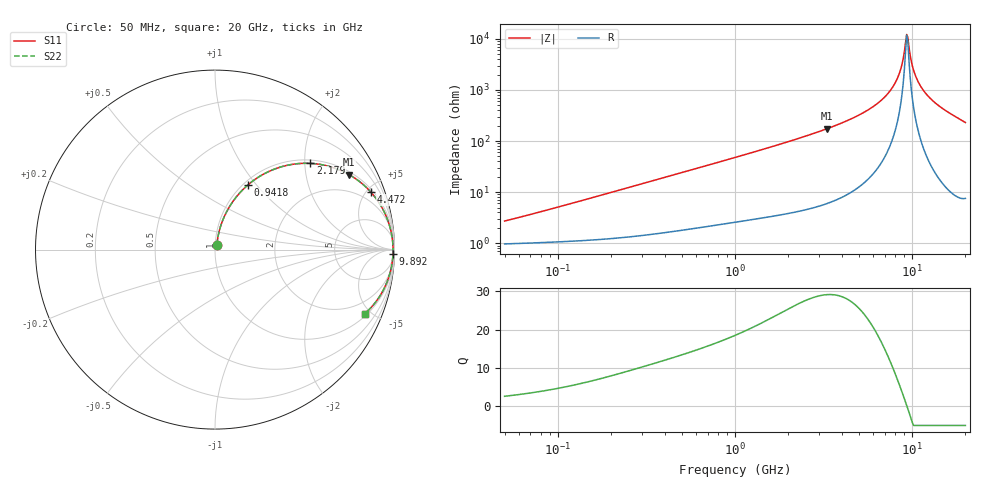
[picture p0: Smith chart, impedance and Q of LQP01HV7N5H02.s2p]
!Murata Part Number: LQP01HV7N5H02
!These Parameters are Measured in Series Mode Connection
!  o--[Z]--o
!Port1  Port2
!  o-------o
!Freq. Start=50[MHz] Stop=20[GHz], 401[Steps]
# Hz S RI R 50
!Freq.(Hz) S11(Real) S11(Imag) S21(Real) S21(Imag) S12(Real) S12(Imag) S22(Real) S22(Imag)
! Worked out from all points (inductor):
!   401 points, 50 MHz to 20 GHz, reference 50 ohm
!   read as one part in series: L = 7.99 nH near 58.96 MHz
!   highest Q = 29.2 at 3.314 GHz (marker M1), where L = 8.39 nH
!   self-resonance near 9.317 GHz
!   S11 on the Smith chart (normalised r, x): 50 MHz: 1.02, +0.05; 941.8 MHz: 1.05, +0.90; 2.179 GHz: 1.08, +2.14; 4.472 GHz: 1.19, +5.33; 9.892 GHz: 22, -71; 20 GHz: 1.15, -4.61
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5e7  0.0102 0.0249  0.9898 -0.0249  0.9898 -0.0249  0.0102 0.0249
1.364002e8  0.0155 0.0657  0.9845 -0.0657  0.9845 -0.0657  0.0155 0.0657
3.721004e8  0.0454 0.1693  0.9546 -0.1693  0.9546 -0.1693  0.0454 0.1693
9.418449e8  0.1811 0.3584  0.8189 -0.3584  0.8189 -0.3584  0.1811 0.3584
1e9  0.1979 0.3723  0.8021 -0.3723  0.8021 -0.3723  0.1979 0.3723
2.179053e9  0.5319 0.4804  0.4681 -0.4804  0.4681 -0.4804  0.5319 0.4804
2.728004e9  0.6502 0.4596  0.3498 -0.4596  0.3498 -0.4596  0.6502 0.4596
3.314454e9  0.7463 0.4183  0.2537 -0.4183  0.2537 -0.4183  0.7463 0.4183
4.472136e9  0.8679 0.3209  0.1321 -0.3209  0.1321 -0.3209  0.8679 0.3209
6.034176e9  0.9485 0.198  0.0515 -0.198  0.0515 -0.198  0.9485 0.198
7.442007e9  0.98 0.1048  0.02 -0.1048  0.02 -0.1048  0.98 0.1048
8.389408e9  0.9892 0.0503  0.0108 -0.0503  0.0108 -0.0503  0.9892 0.0503
8.774992e9  0.9911 0.0297  0.00893 -0.0297  0.00893 -0.0297  0.9911 0.0297
9.178299e9  0.992 0.00899  0.00798 -0.00899  0.00798 -0.00899  0.992 0.00899
9.316812e9  0.9921 0.00208  0.00786 -0.00208  0.00786 -0.00208  0.9921 0.00208
9.600142e9  0.9921 -0.0118  0.00791 0.0118  0.00791 0.0118  0.9921 -0.0118
9.892087e9  0.9916 -0.0256  0.00836 0.0256  0.00836 0.0256  0.9916 -0.0256
1.019291e10  0.9908 -0.0395  0.00921 0.0395  0.00921 0.0395  0.9908 -0.0395
1.066139e10  0.9888 -0.0604  0.0112 0.0604  0.0112 0.0604  0.9888 -0.0604
1.220001e10  0.977 -0.1232  0.023 0.1232  0.023 0.1232  0.977 -0.1232
1.482269e10  0.9435 -0.2144  0.0565 0.2144  0.0565 0.2144  0.9435 -0.2144
2e10  0.8338 -0.3563  0.1662 0.3563  0.1662 0.3563  0.8338 -0.3563
